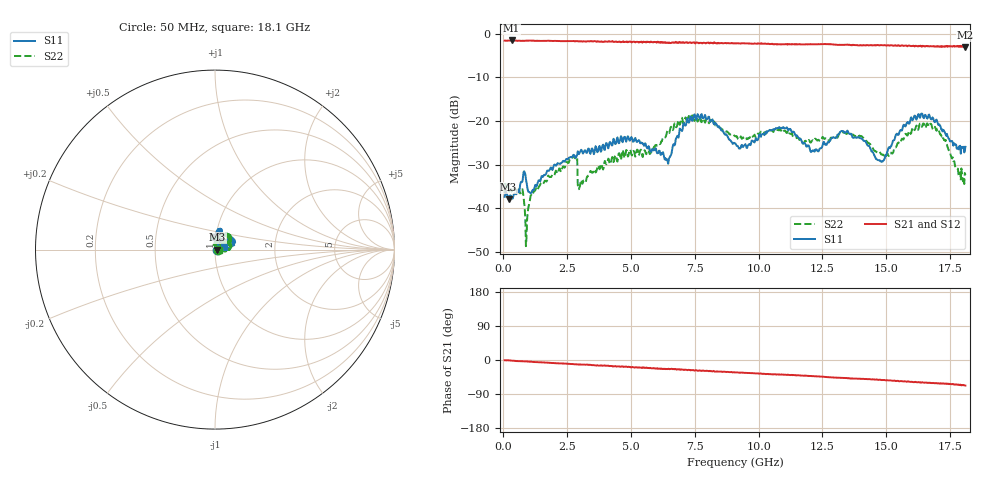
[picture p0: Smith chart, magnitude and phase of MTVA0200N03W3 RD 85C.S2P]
! Network Analyzer HP8720D.06.14 Serial No. US36140669
! 17 Jan 2005  12:11:57
! Frequency  S11  S21  S12  S22
# HZ  S  DB R 50
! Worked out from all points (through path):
!   801 points, 50 MHz to 18.1 GHz, reference 50 ohm
!   highest |S21| = -1.57 dB at 320.8 MHz (marker M1); lowest = -3.1 dB at 18.1 GHz (marker M2)
!   group delay of S21, straight-line fit = 9.8 ps
!   lowest |S11| = -37.9 dB at 207.9 MHz (marker M3), VSWR 1.03, Z = 51.3 + j0.0542 ohm
!   |S11| at or under -10 dB: start of sweep to end of sweep
!   |S22| runs from -48.7 to -18.7 dB; largest |S21 - S12| = 0.024
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5e7  -37.40 -15.3  -1.60 -0.8  -1.60 -1.1  -36.54 0.7
2.079375e8  -37.95 2.4  -1.58 -0.9  -1.58 -1.2  -35.80 -4.4
3.2075e8  -37.56 4.5  -1.57 -1.6  -1.57 -2.0  -35.66 -6.1
7.043125e8  -33.93 30.8  -1.66 -3.2  -1.66 -3.6  -36.10 -2.1
9.299375e8  -34.85 6.7  -1.62 -4.0  -1.61 -4.1  -42.68 103.6
1.155562e9  -35.76 38.6  -1.62 -4.9  -1.61 -5.3  -36.25 66.9
2.689812e9  -28.31 61.1  -1.70 -10.6  -1.70 -10.9  -28.68 82.6
3.073375e9  -26.77 62.0  -1.77 -12.3  -1.73 -12.4  -33.98 83.3
4.946062e9  -24.53 63.7  -1.85 -18.3  -1.85 -19.1  -26.75 78.6
6.074188e9  -27.34 66.8  -1.99 -23.4  -1.97 -23.2  -25.48 77.9
6.45775e9  -29.81 64.2  -2.16 -23.3  -2.19 -23.7  -22.27 72.9
6.99925e9  -22.33 75.4  -2.04 -25.6  -2.09 -26.5  -19.27 56.9
7.54075e9  -19.59 71.1  -2.08 -26.6  -1.95 -28.1  -18.73 46.5
9.075e9  -25.16 86.2  -2.24 -32.6  -2.20 -33.0  -23.49 26.1
1.103794e10  -21.71 102.0  -2.44 -38.8  -2.41 -39.4  -22.27 21.5
1.209838e10  -26.95 76.4  -2.42 -42.5  -2.42 -42.7  -24.53 36.6
1.327162e10  -22.33 51.3  -2.58 -47.1  -2.58 -47.6  -22.53 41.5
1.476075e10  -29.21 35.9  -2.65 -52.1  -2.65 -52.6  -27.25 27.1
1.509919e10  -26.03 12.1  -2.71 -54.2  -2.63 -54.3  -28.05 39.7
1.604681e10  -19.72 19.5  -2.79 -58.0  -2.91 -58.1  -21.51 28.9
1.667856e10  -18.53 31.2  -2.96 -60.4  -2.83 -60.7  -21.27 12.1
1.81e10  -25.93 19.3  -3.13 -67.5  -3.03 -68.3  -32.35 -10.9
